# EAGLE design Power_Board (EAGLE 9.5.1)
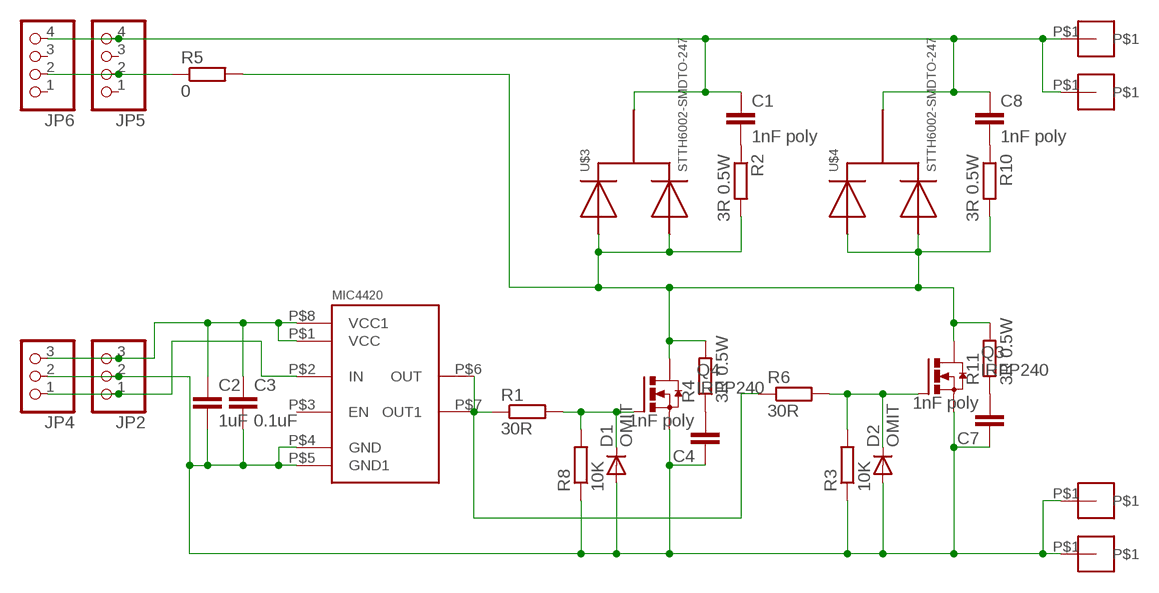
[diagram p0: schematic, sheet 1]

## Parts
C1  1nF poly  C-EU050-045X075  [C050-045X075]
C2  1uF  C-EUC1206  [C1206]
C3  0.1uF  C-EUC1206  [C1206]
C4  1nF poly  C-EU050-045X075  [C050-045X075]
C7  1nF poly  C-EU050-045X075  [C050-045X075]
C8  1nF poly  C-EU050-045X075  [C050-045X075]
D1  OMIT  DIODE-SOD123  [SOD123]
D2  OMIT  DIODE-SOD123  [SOD123]
JP2  PINHD-1X3  [1X03]
JP4  PINHD-1X3  [1X03]
JP5  PINHD-1X4  [1X04]
JP6  PINHD-1X4  [1X04]
MIC4420  IXDD414CI  [SOIC8]
Q3  IRFP240  [TO247BV]
Q4  IRFP240  [TO247BV]
R1  30R  R-EU_R1206  [R1206]
R2  3R 0.5W  R-EU_0309/V  [0309V]
R3  10K  R-EU_R1206  [R1206]
R4  3R 0.5W  R-EU_0309/V  [0309V]
R5  0  R-EU_R1206  [R1206]
R6  30R  R-EU_R1206  [R1206]
R8  10K  R-EU_R1206  [R1206]
R10  3R 0.5W  R-EU_0309/V  [0309V]
R11  3R 0.5W  R-EU_0309/V  [0309V]
U$1  BIG_PINHEADX1M4  [M4_PINHEAD]
U$2  BIG_PINHEADX1M4  [M4_PINHEAD]
U$3  STTH6002-SMDTO-247  [TO-247]
U$4  STTH6002-SMDTO-247  [TO-247]
U$5  BIG_PINHEADX1M4  [M4_PINHEAD]
U$6  BIG_PINHEADX1M4  [M4_PINHEAD]

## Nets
N$1: D1.C Q4.G R1.2 R8.2
N$2: C1.1 C8.1 JP5.4 JP6.4 U$3.D(K) U$4.D(K) U$5.P$1 U$6.P$1
N$3: JP2.1 JP4.1 MIC4420.P$2(IN)
N$4: JP5.2 JP6.2 R5.1
N$5: C1.2 R2.1
N$9: C4.2 R4.1
N$10: C7.2 R11.1
N$11: D2.C Q3.G R3.2 R6.2
N$14: C8.2 R10.1
N$17: MIC4420.P$6(OUT) MIC4420.P$7(OUT1) R1.1 R6.1
N$18: Q3.D Q4.D R2.2 R4.2 R5.2 R10.2 R11.2 U$3.G(A1) U$3.S(A2) U$4.G(A1) U$4.S(A2)
N$19: C2.2 C3.2 C4.1 C7.1 D1.A D2.A JP2.2 JP4.2 MIC4420.P$4(GND) MIC4420.P$5(GND1) Q3.S Q4.S R3.1 R8.1 U$1.P$1 U$2.P$1
N$21: C2.1 C3.1 JP2.3 JP4.3 MIC4420.P$1(VCC) MIC4420.P$8(VCC1)
Unconnected: JP5.1 JP5.3 JP6.1 JP6.3 MIC4420.P$3(EN)

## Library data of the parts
C1-C4 C7 C8 = resistor:C-EU: CAPACITOR, European symbol
D1 D2 = diode:DIODE-: DIODE
JP2 JP4 = pinhead:PINHD-1X3: PIN HEADER
JP5 JP6 = pinhead:PINHD-1X4: PIN HEADER
MIC4420 = Ians parts:IXDD414CI: IXYS 14A MOSFET driver
Q3 Q4 = transistor-power:IRFP240: HEXFET Power MosFet Source: http://www.irf.com/
R1-R6 R8 R10 R11 = resistor:R-EU_: RESISTOR, European symbol
U$1 U$2 U$5 U$6 = Ians parts:BIG_PINHEADX1
U$3 U$4 = Ians parts:STTH6002-SMD

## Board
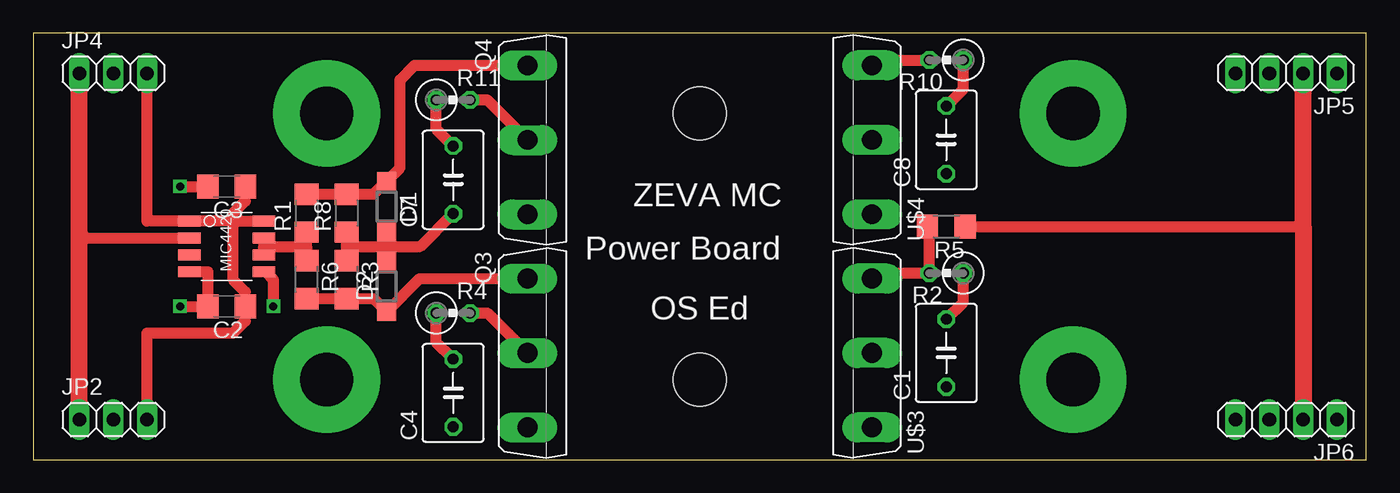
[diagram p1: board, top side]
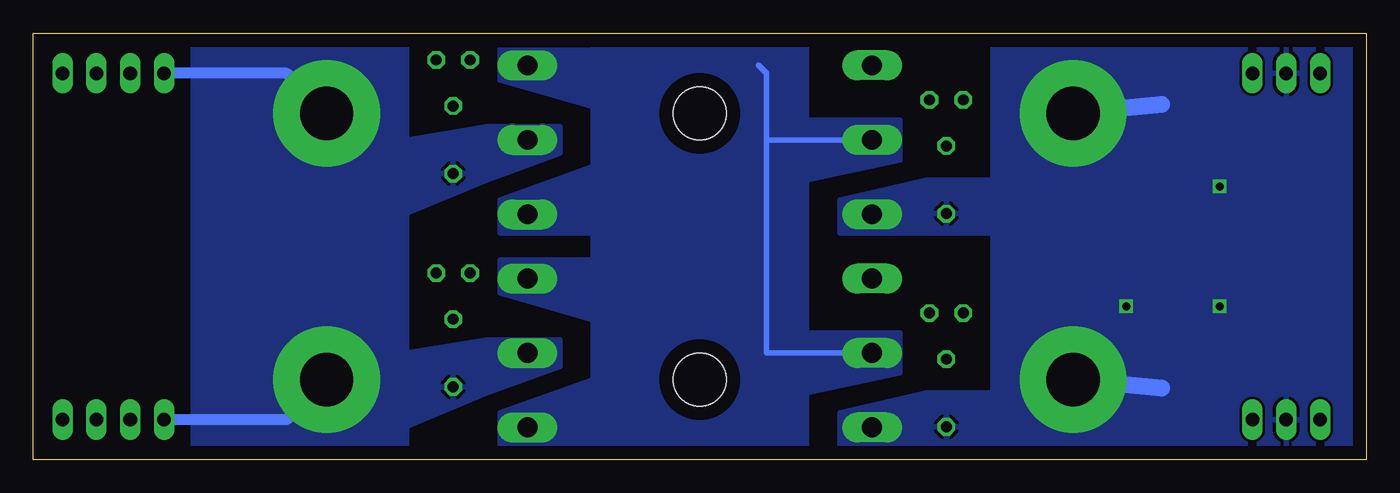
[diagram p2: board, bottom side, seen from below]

Size 100 x 32 mm. Coordinates in mm from the lower left corner, seen from the top.
Outline: 0,0 100,0 100,32 0,32 0,0
Copper layers (1*16): Top 0.035mm / dielectric 1.5mm / Bottom 0.035mm
Design rules "default": minimum track width 10mil, minimum drill 24mil, track to track 8mil, track to pad 8mil, pad to pad 8mil, via to via 8mil, smd to smd 8mil, copper to edge 40mil, drill to drill 8mil, minimum pad ring 10mil, minimum via ring 8mil, stop-mask expansion 4mil, vias tented up to drill 0mil, thermal gap 10mil
Holes 4 mm at 50,26 50,6

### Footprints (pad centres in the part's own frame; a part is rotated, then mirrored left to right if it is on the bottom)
C050-045X075 = drill 0.813 octagon: 1 -2.54,0; 2 2.54,0
C1206 = smd 1.6 x 1.8: 1 -1.4,0; 2 1.4,0
SOD123 = smd 1.4 x 1.4: A 1.9,0; C -1.9,0
1X03 = drill 1.016 long: 1 -2.54,0; 2 0,0; 3 2.54,0
1X04 = drill 1.016 long: 1 -3.81,0; 2 -1.27,0; 3 1.27,0; 4 3.81,0
SOIC8 = smd 1.676 x 0.813: P$1 -2.794,1.905; P$2 -2.794,0.635; P$3 -2.794,-0.635; P$4 -2.794,-1.905; P$5 2.794,-1.905; P$6 2.794,-0.635; P$7 2.794,0.635; P$8 2.794,1.905
TO247BV = drill 1.499 long: D 0,-2.921; G -5.588,-2.921; S 5.588,-2.921
R1206 = smd 1.6 x 1.803: 1 -1.422,0; 2 1.422,0
0309V = drill 0.813 octagon: 1 -1.27,0; 2 1.27,0
M4_PINHEAD = drill 4 pad 8: P$1 0,0
TO-247 = drill 1.499 long: D 0,-2.921; G -5.588,-2.921; S 5.588,-2.921

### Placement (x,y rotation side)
C1  68.5,8 90 top
C2  14.5,11.5 180 top
C3  14.5,20.5 180 top
C4  31.5,5 90 top
C7  31.5,21 90 top
C8  68.5,24 90 top
D1  26.5,19 270 top
D2  26.5,13 90 top
JP2  6,3 0 top
JP4  6,29 0 top
JP5  94,29 180 top
JP6  94,3 180 top
MIC4420  14.5,16 0 top
Q3  40,8 270 top
Q4  40,24 270 top
R1  20.5,18.5 90 top
R2  68.5,14 180 top
R3  23.5,13.5 270 top
R4  31.5,11 0 top
R5  68.5,17.5 180 top
R6  20.5,13.5 270 top
R8  23.5,18.5 90 top
R10  68.5,30 180 top
R11  31.5,27 0 top
U$1  22,6 0 top
U$2  22,26 0 top
U$3  60,8 90 top
U$4  60,24 90 top
U$5  78,6 0 top
U$6  78,26 0 top

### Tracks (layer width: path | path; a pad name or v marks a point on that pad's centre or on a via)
N$1
  Top 0.813: R1.2 R8.2 25.52,19.92 D1.C 27.5,21.9 27.5,28.5 28.59,29.59 Q4.G
N$2
  Bottom 0.813: U$6.P$1 81,29 JP5.4 | U$5.P$1 81,3 JP6.4
  pour Bottom: 72,33 88,33 88,-1 72,-1
  pour Bottom (no thermals): 66,21 60.5,23 60.5,25 66,25
  pour Bottom: 72,18.5 66,21 66,25 72,24
  pour Bottom (no thermals): 66,5 60.5,7 60.5,9 66,9
  pour Bottom: 72,2.5 66,5 66,9 72,8
N$3
  Top 0.813: MIC4420.P$2 3.46,16.64 3.46,17
  Top 1.27: JP2.1 3.46,17 JP4.1
N$4
  Top 0.813: R5.1 95.27,17.5
  Top 1.27: JP6.2 95.27,17.5 JP5.2
N$5
  Top 0.813: R2.1 69.77,11.81 C1.2
N$9
  Top 0.813: C4.2 30.23,8.81 R4.1
N$10
  Top 0.813: C7.2 30.23,24.81 R11.1
N$11
  Top 0.813: R6.2 R3.2 25.52,12.08 D2.C 28.99,13.59 Q3.G
N$14
  Top 0.813: C8.2 69.77,27.81 R10.1
N$17
  Top 0.813: 20.5,16 R6.1 | 20.5,16 R1.1 | MIC4420.P$7 MIC4420.P$6 17.29,16 20.5,16
N$18
  Top 0.813: Q4.D 34.08,27 R11.2 | Q3.D 34.08,11 R4.2 | R10.2 63.33,30 U$4.S | U$3.S 63.33,14 R2.2 67.23,16.85 R5.2
  Bottom 0.406: 45,24 Q4.D | 45,24 45,29 45.59,29.59 | Q3.D 45,8 45,24
  pour Bottom: 42,33 58,33 58,-1 42,-1
  pour Bottom (no thermals): 42,5 35,6.5 35,9.5 42,9.5
  pour Bottom (no thermals): 42,21 35,22.5 35,25.5 42,25.5
  pour Bottom (no thermals): 65,28.5 58,26.5 58,31 65,31
  pour Bottom (no thermals): 65,12.5 58,10.5 58,15 65,15
  pour Bottom (no thermals): 65,17 58,17 58,22 65,19.5
  pour Bottom (no thermals): 65,1 58,1 58,6 65,3.5
N$19  (via drill 0.6)
  Top 0.406: 17.41,14.1 18,13.5
  Top 0.813: R3.1 23.5,16 | 23.5,16 R8.1 | 26.5,16 D1.A | 26.5,16 D2.A | 23.5,16 26.5,16 | C7.1 29.04,16 26.5,16 | MIC4420.P$4 13.1,14.1 C2.2 v11,11.5 | v11,20.5 C3.2 | v18,11.5 18,13.5 17.5,14.1 17.41,14.1 MIC4420.P$5
  Bottom 1.27: 15.35,26.65 U$2.P$1 | 15.35,5.35 U$1.P$1
  pour Bottom: -1,33 28,33 28,-1 -1,-1
  pour Bottom: 28,5 33,5 33,-1 28,-1
  pour Bottom (no thermals): 33,5 39.5,3.5 39.5,-0.5 33,-0.5
  pour Bottom: 28,21 33,21 33,17 28,17
  pour Bottom (no thermals): 33,21 39.5,19.5 39.5,17 33,17
N$21
  Top 0.813: 15,17.91 MIC4420.P$1 8.54,17.91 JP4.3 | 15,17.91 MIC4420.P$8 | 15,17.91 15,13.5 15.9,12.6 C2.1 15.9,10.4 15,9.5 8.54,9.5 JP2.3 | C3.1 15.9,19.4 15,18.5 15,17.91

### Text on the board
tPlace: ZEVA MC | Power Board | OS Ed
